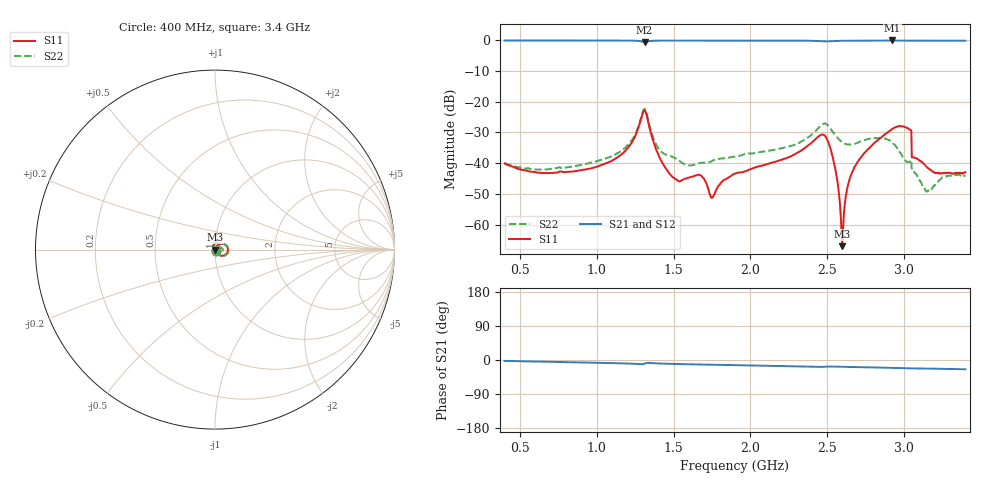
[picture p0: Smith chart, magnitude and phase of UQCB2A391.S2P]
!  Part Number  UQCB2A391	Mounting Orientation: Vertical
!  Description: RF capacitors
!  Application: Coupling, Bypass, Tuning, DC Block
!  Filters, Matching
# GHZ S DB R 50
! Freq  |S11|  S11 Ph  |S21|  S21 Ph  |S12|  S12 Ph  |S22|  S22 Ph
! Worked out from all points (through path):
!   801 points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, 400 MHz to 3.4 GHz, reference 50 ohm
!   highest |S21| = -0.06 dB at 2.924 GHz (marker M1); lowest = -0.7 dB at 1.311 GHz (marker M2)
!   group delay of S21, straight-line fit = 19.9 ps
!   lowest |S11| = -67.0 dB at 2.598 GHz (marker M3), VSWR 1.00, Z = 50 - j0.0295 ohm
!   |S11| at or under -10 dB: start of sweep to end of sweep
!   |S22| runs from -49.2 to -22.3 dB; largest |S21 - S12| = 0.0012
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0.4  -40.09 -46.9  -0.07 -2.4  -0.06 -2.4  -39.93 -45.6
0.903  -42.18 23.9  -0.07 -6.5  -0.08 -6.5  -40.51 18.9
1.173  -36.59 54.2  -0.10 -8.9  -0.09 -8.9  -35.50 43.4
1.311  -22.81 -3.5  -0.68 -9.5  -0.68 -9.5  -22.34 -4.1
1.401  -37.27 -58.8  -0.12 -9.2  -0.12 -9.2  -35.14 -46.0
1.525  -45.56 -16.8  -0.10 -10.6  -0.10 -10.6  -38.81 -26.6
1.683  -44.20 2.4  -0.10 -11.9  -0.09 -11.9  -39.84 3.7
1.75  -51.22 26.8  -0.11 -12.4  -0.11 -12.4  -39.29 11.8
1.9  -43.34 61.9  -0.10 -13.6  -0.10 -13.6  -37.86 16.4
2.403  -33.16 62.7  -0.18 -17.9  -0.18 -17.9  -30.54 22.7
2.47  -30.66 25.3  -0.34 -18.2  -0.34 -18.2  -27.30 3.1
2.508  -33.17 -13.1  -0.35 -17.4  -0.35 -17.4  -27.80 -20.8
2.553  -41.80 -43.2  -0.23 -17.4  -0.22 -17.4  -30.89 -32.1
2.598  -66.98 -138.7  -0.17 -17.9  -0.17 -17.9  -33.13 -28.4
2.635  -47.17 132.1  -0.15 -18.3  -0.15 -18.3  -33.94 -20.8
2.676  -41.37 124.6  -0.14 -18.7  -0.14 -18.7  -33.73 -13.4
2.901  -29.71 95.1  -0.08 -20.4  -0.07 -20.4  -32.47 -33.4
2.924  -28.88 89.7  -0.06 -20.7  -0.06 -20.7  -33.27 -37.8
3.033  -28.87 57.8  -0.12 -22.1  -0.12 -22.1  -39.61 -4.6
3.066  -38.15 -59.0  -0.14 -22.2  -0.14 -22.2  -42.96 18.0
3.149  -41.23 -67.8  -0.15 -22.6  -0.15 -22.6  -49.24 32.8
3.4  -42.94 -35.1  -0.16 -24.5  -0.16 -24.5  -44.22 20.1
